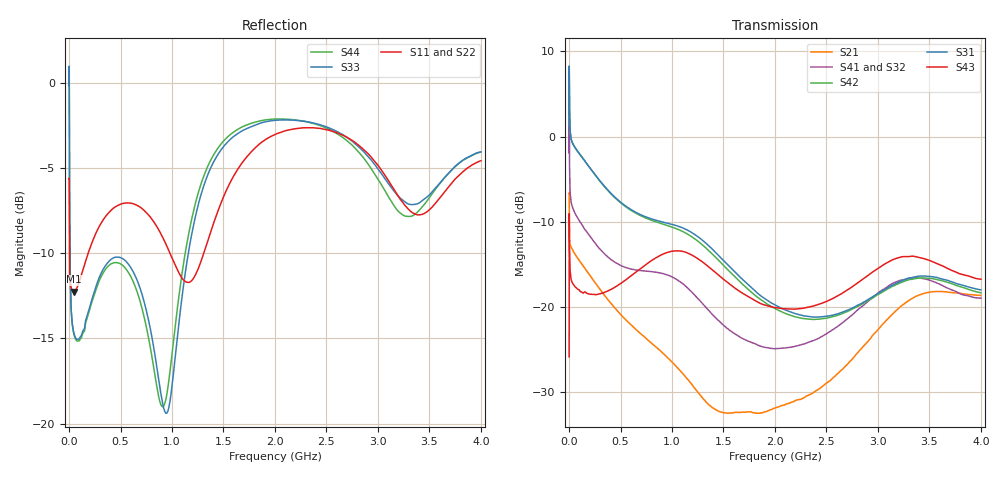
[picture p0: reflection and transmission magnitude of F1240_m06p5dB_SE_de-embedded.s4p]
! Integrated Device Technology
! Corporate Headquarters
! 6024 Silver Creek Valley Road
! San Jose, CA 95138  USA
! Phone:  1-408-284-8200
! Toll Free:  1-800-223-1366
! Webpage:  http://www.idt.com/
! Timing and RF Division
! 515 Groton Road, Suite 102
! Westford, MA 01886-6024
! Device:  F1240
! Description: Dual Intermediate Frequency Digital Variable Gain Amplifier
! Frequency:  10.0 -  500.00 MHz
! Package:  5x5 mm QFN Plastic Package: 32 pin
! Ports:  8 RF, 20 DC
!  Pin  1  = GA3 / Data  Pin 17  = RF OUT_B+
!  Pin  2  = GA4 / CLK  Pin 18  = RF OUT_B-
!  Pin  3  = GA5  Pin 19  = STBY_B
!  Pin  4  = VMODE  Pin 20  = Ground
!  Pin  5  = No Connect  Pin 21  = Ground
!  Pin  6  = GB5  Pin 22  = STB_A
!  Pin  7  = GB4  Pin 23  = RF OUT_A-  = Port 4
!  Pin  8  = GB3  Pin 24  = RF OUT_A+  = Port 3
!  Pin  9  = GB2  Pin 25  = GA0
!  Pin 10  = GB1  Pin 26  = ISET_A
!  Pin 11  = RF IN_B+  Pin 27  = VCC
!  Pin 12  = RF IN_B-  Pin 28  = Ground
!  Pin 13  = Ground  Pin 29  = RF IN_A-  = Port 2
!  Pin 14  = VCC  Pin 30  = RF IN_A+  = Port 1
!  Pin 15  = ISET_B  Pin 31  = GA1
!  Pin 16  = GB0  Pin 32  = GA2 / CSb
! Gain  = +19.5 dB
! State  = 1
! Voltage  = +5.00 V
! Current  = 85.292 mA (one channel only)
! Temperture  =  +25 C
! Test Date  =  2017-10-18
! Board  =  EB4031
! Data:  The device was measured on a custom evaluation board which has
!  individual transmission lines to the RF pins.  Data was collected
!  using a calibrated network analyzer.  The evaluation board was
!  de-embedded using Automatic Fixture Removal.
!  The reference plane is the edge of the package pin.
!  Only Channel A was measured.
!  This data is in single-ended operation.  If your needs are balanced
!  or differential S-parameters then this file needs to be used a
!  linear simulator.
! File Date:  2017-11-10  MJV
! Note:
!  Integrated Device Technology supplies this data as a sample of measured
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# Hz S dB R 100
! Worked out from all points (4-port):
!   410 points, 500 kHz to 4 GHz, reference 100 ohm
!   strongest paths, dB at 500 kHz, 930 MHz, 1.96 GHz, 2.98 GHz, 4 GHz:
!     S43: -25.8, -13.7, -19.9, -15.6, -16.7
!     S31: 1.4, -10.1, -19.5, -18.5, -18.0
!     S42: 1.4, -10.3, -19.9, -18.7, -18.3
!     S41: -1.9, -16.1, -24.8, -18.6, -18.9
!     S32: -1.9, -16.3, -24.7, -18.8, -19.3
!     S21: -6.6, -25.6, -32.0, -22.9, -18.6
!   lowest |S11| = -12.2 dB at 50 MHz (marker M1), VSWR 1.65, Z = 138 - j45.3 ohm
!   |S11| at or under -10 dB: 2.938 MHz to 185.2 MHz (182.3 MHz wide, 194 % of centre); 980.2 MHz to 1.308 GHz (327.5 MHz wide, 28.6 % of centre)
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500000  -5.61 -5.6  -6.60 -5.8  -31.40 78.3  -34.62 77.0
        -6.61 -5.8  -5.61 -5.6  -34.56 76.0  -31.41 79.4
        1.37 -110.2  -1.91 -112.3  -0.14 0.1  -25.82 -39.4
        -1.93 -111.2  1.37 -109.1  -25.82 -39.4  -0.15 2.4
2000000  -8.24 -29.1  -9.57 -29.4  -23.11 21.1  -27.01 5.4
         -9.57 -29.4  -8.22 -29.2  -26.97 5.1  -23.09 21.3
         7.55 176.4  3.60 160.7  -0.29 -54.2  -9.03 -145.4
         3.56 161.0  7.56 176.7  -9.04 -145.5  -0.33 -53.9
4000000  -10.87 -22.5  -12.07 -19.2  -23.94 4.6  -30.00 -11.4
         -12.07 -19.2  -10.87 -22.7  -29.97 -11.6  -23.94 4.7
         4.02 156.3  -2.05 140.0  -4.80 -87.5  -11.94 172.4
         -2.08 140.2  4.03 156.5  -11.95 172.4  -4.84 -87.5
5e7  -12.25 -39.3  -13.63 -23.4  -25.16 -17.0  -32.63 -19.9
     -13.63 -23.4  -12.21 -39.8  -32.62 -19.8  -25.13 -17.1
     -1.16 152.4  -8.80 142.3  -14.76 -163.0  -17.51 152.4
     -8.79 142.4  -1.11 152.2  -17.47 152.3  -14.83 -163.5
5.2e8  -7.07 -148.1  -21.09 -128.4  -28.64 -104.5  -36.60 -91.5
       -21.10 -128.2  -7.03 -149.0  -36.72 -89.6  -28.93 -104.5
       -7.88 25.7  -15.32 -26.1  -10.31 -174.6  -17.16 8.9
       -15.22 -27.5  -7.95 24.1  -17.07 8.6  -10.71 -175.2
2.91e9  -4.19 101.1  -23.93 -29.5  -28.28 -158.0  -30.54 -143.3
        -23.92 -29.6  -3.97 101.8  -31.17 -130.1  -29.68 -150.6
        -19.07 -73.3  -19.55 -155.0  -4.36 94.1  -17.03 -91.2
        -19.25 -166.7  -19.19 -70.0  -16.22 -89.4  -4.81 86.7
4e9  -4.56 -127.8  -18.64 118.6  -27.18 -28.5  -28.17 -13.1
     -18.63 118.6  -4.31 -126.5  -28.76 0.8  -29.06 -19.0
     -17.97 48.7  -19.27 -47.3  -4.04 -133.2  -18.08 62.5
     -18.95 -61.7  -18.32 54.8  -16.73 55.7  -4.05 -143.1
